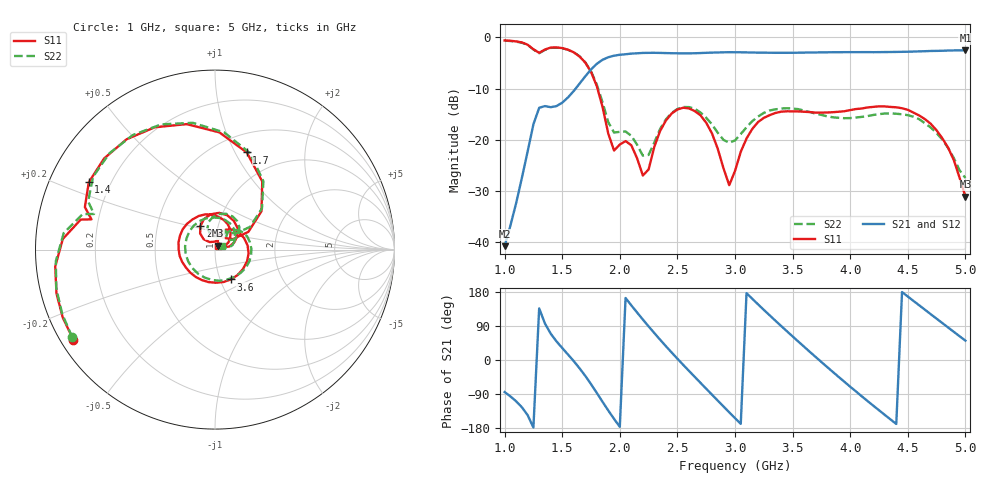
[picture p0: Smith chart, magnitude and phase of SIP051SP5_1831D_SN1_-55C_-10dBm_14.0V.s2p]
# GHz  S  dB  R  50
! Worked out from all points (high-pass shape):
!   81 points, 1 GHz to 5 GHz, reference 50 ohm
!   highest |S21| = -2.50 dB at 5 GHz (marker M1); lowest = -40.8 dB at 1 GHz (marker M2)
!   |S21| within 3 dB of the highest: 1.784 GHz to end of sweep
!   lowest |S11| = -31.1 dB at 5 GHz (marker M3), VSWR 1.06, Z = 51.8 + j2.23 ohm
!   |S11| at or under -10 dB: 1.806 GHz to end of sweep
!   |S22| runs from -27.4 to -0.6 dB; largest |S21 - S12| = 0.0019
!   S11 on the Smith chart (normalised r, x): 1 GHz: 0.04, -0.29; 1.4 GHz: 0.12, +0.25; 1.7 GHz: 0.70, +1.12; 2.4 GHz: 0.82, +0.22; 3.6 GHz: 1.12, -0.39; 5 GHz: 1.04, +0.04
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1  -0.58 -147.5  -40.77 -84.6  -41.26 -85.7  -0.60 -148.4
1.25  -2.31 167.4  -16.96 -178.2  -16.97 -178.4  -2.34 165.0
1.4  -1.97 151.9  -13.62 69.6  -13.61 69.5  -2.03 149.1
1.55  -2.39 116.3  -11.71 14.6  -11.70 14.7  -2.39 113.2
1.7  -4.89 71.9  -7.59 -41.8  -7.59 -41.7  -4.85 70.1
1.85  -13.54 28.0  -4.36 -110.3  -4.35 -110.2  -12.65 33.0
2  -20.92 76.1  -3.38 -176.3  -3.38 -176.3  -18.44 63.4
2.2  -26.96 85.8  -3.02 106.8  -3.02 106.9  -23.09 72.6
2.35  -18.25 132.7  -3.01 53.5  -3.00 53.6  -17.86 109.1
2.4  -16.22 121.8  -3.04 36.5  -3.04 36.6  -16.00 102.8
2.55  -13.72 83.5  -3.11 -12.7  -3.10 -12.7  -13.59 72.6
2.75  -16.65 31.8  -2.99 -75.8  -2.99 -75.8  -15.69 35.3
2.95  -28.86 43.4  -2.87 -138.1  -2.88 -138.1  -20.57 41.6
3  -26.08 75.0  -2.89 -153.4  -2.87 -153.4  -20.11 50.0
3.15  -17.87 60.8  -2.93 161.6  -2.93 161.6  -16.34 46.8
3.35  -14.76 7.4  -3.00 103.9  -2.99 104.0  -14.05 12.4
3.6  -14.51 -62.1  -2.95 35.0  -2.96 34.9  -14.29 -42.3
3.7  -14.67 -88.6  -2.92 8.0  -2.92 8.0  -14.88 -68.1
4.05  -13.98 -169.9  -2.86 -83.0  -2.86 -83.1  -15.63 -171.3
4.35  -13.57 126.7  -2.84 -156.8  -2.85 -156.8  -14.84 106.5
4.7  -16.88 54.5  -2.63 120.7  -2.64 120.7  -17.60 30.9
5  -31.10 50.6  -2.50 51.1  -2.50 51.0  -27.44 29.8
